FUNCTION_BLOCK FB_LN_IED_LD1_LEDGGIO4 EXTENDS FB_AcsiCommonLogicalNodeClass
VAR_INPUT
	NamPlt: FB_DO_IED_LD1_LEDGGIO4_NamPlt := (sClass:='LPL', bLinkResult:=THIS^.AddDataToContainer(ipData:=NamPlt));
	Beh: FB_DO_IED_LD1_LEDGGIO4_Beh := (sClass:='ENS', bLinkResult:=THIS^.AddDataToContainer(ipData:=Beh));
	Health: FB_DO_IED_LD1_LEDGGIO4_Health := (sClass:='ENS', bLinkResult:=THIS^.AddDataToContainer(ipData:=Health));
	Mod_: FB_DO_IED_LD1_LEDGGIO4_Mod := (sObjectName:='Mod', sClass:='ENC', bLinkResult:=THIS^.AddDataToContainer(ipData:=Mod_));
	SPCSO1: FB_DO_IED_LD1_LEDGGIO4_SPCSO1 := (sClass:='SPC', bLinkResult:=THIS^.AddDataToContainer(ipData:=SPCSO1));
END_VAR
VAR
END_VAR

END_FUNCTION_BLOCK
